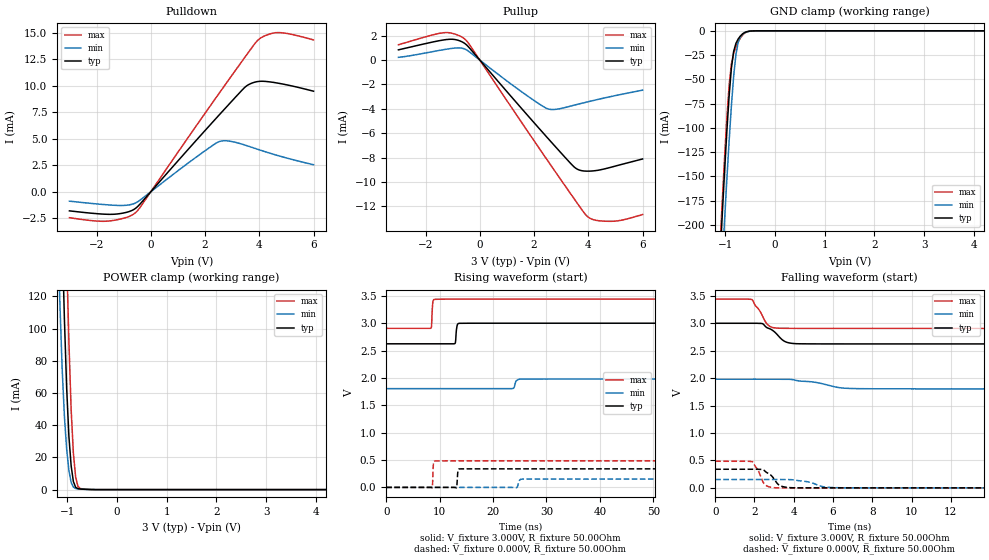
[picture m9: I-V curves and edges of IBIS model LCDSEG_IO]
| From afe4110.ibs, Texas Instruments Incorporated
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[Model]   LCDSEG_IO
Model_type   I/O
Vinl = 0.9V
Vinh = 2.1V
Vmeas = 1.500V
Cref = 25pF
|   typ   min   max
|   (NOM)   (WEAK)   (FAST)
C_comp   0.9946pF   0.9809pF   1.0463pF
[Model Spec]
Vinl   0.9V   0.594V   1.032V
Vinh   2.1V   1.386V   2.408V
[Voltage Range]   3.000V   1.980V   3.440V
[Temperature Range]   27.0   85.0   0.0
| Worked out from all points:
|   slope of the pulldown table from 0 to 0.45 V, typ, clamps not added: 342 ohm
|   slope of the pullup table from 0 to 0.45 V, typ, clamps not added: 385 ohm
|   GND clamp passes 1 mA (typ) near -0.57 V on its own axis
|   POWER clamp passes 1 mA (typ) near -0.81 V on its own axis
|   falling waveform, V_fixture 3.000V, R_fixture 50.00Ohm: 20-80 % time 803ps typ, 1.73ns min, 559ps max; typ from 3 V to 2.62 V
|   rising waveform, V_fixture 3.000V, R_fixture 50.00Ohm: 20-80 % time 203ps typ, 344ps min, 161ps max; typ from 2.62 V to 3 V
|   rising waveform, V_fixture 0.000V, R_fixture 50.00Ohm: 20-80 % time 139ps typ, 288ps min, 109ps max; typ from 0 V to 0.339 V
|   falling waveform, V_fixture 0.000V, R_fixture 50.00Ohm: 20-80 % time 535ps typ, 900ps min, 399ps max; typ from 0.339 V to 0 V
[Pulldown]
|   Voltage   I(typ)   I(min)   I(max)
-3V       -1.798mA   -884uA     -2.443mA
-1.598V   -2.122mA   -1.23mA    -2.769mA
-1.01V    -2.002mA   -1.288mA   -2.501mA
-603mV    -1.633mA   -1.101mA   -2.05mA
-376.9mV  -1.1mA     -754.7uA   -1.404mA
2.472V    7.106mA    4.676mA    9.115mA
2.834V    8.118mA    4.795mA    10.42mA
3.467V    9.847mA    4.407mA    12.67mA
3.965V    10.4mA     3.986mA    14.33mA
4.281V    10.39mA    3.726mA    14.78mA
4.688V    10.24mA    3.412mA    15.01mA
6V        9.481mA    2.549mA    14.32mA
[GND Clamp]
|   Voltage   I(typ)   I(min)   I(max)
-3V       -2.438A    -2.419A    -2.47A
-1.101V   -232.4mA   -281.6mA   -219.7mA
-1.055V   -187.1mA   -237.2mA   -173.3mA
-1.01V    -143.6mA   -194mA     -129.3mA
-964.8mV  -102.9mA   -152.5mA   -89.25mA
-919.6mV  -66.79mA   -113.3mA   -56.1mA
-874.4mV  -38.47mA   -77.46mA   -34.26mA
-829.1mV  -21.25mA   -47.02mA   -23.15mA
-783.9mV  -13.01mA   -24.69mA   -16.57mA
-738.7mV  -8.486mA   -11.97mA   -11.47mA
-603mV    -1.62mA    -1.923mA   -2.206mA
6V        0A         0A         0A
[Pullup]
|   Voltage   I(typ)   I(min)   I(max)
-3V       837uA      223uA      1.256mA
-1.327V   1.649mA    853.7uA    2.241mA
-919.6mV  1.683mA    980.9uA    2.13mA
-603mV    1.431mA    941.8uA    1.805mA
-376.9mV  979.2uA    661uA      1.255mA
2.472V    -6.315mA   -3.964mA   -8.145mA
2.834V    -7.212mA   -4.031mA   -9.311mA
3.513V    -8.822mA   -3.68mA    -11.47mA
3.965V    -9.104mA   -3.432mA   -12.81mA
4.281V    -9.056mA   -3.266mA   -13.13mA
4.869V    -8.765mA   -2.973mA   -13.21mA
6V        -8.106mA   -2.468mA   -12.66mA
[POWER Clamp]
|   Voltage   I(typ)   I(min)   I(max)
-3V       3.094A     2.811A     3.32A
-1.191V   277.9mA    163.8mA    401.2mA
-1.146V   216.5mA    115.6mA    333.9mA
-1.101V   158.6mA    75.42mA    268.1mA
-1.055V   106.3mA    45.57mA    204.8mA
-1.01V    63.3mA     25.24mA    145.1mA
-964.8mV  33.18mA    11.91mA    91.89mA
-919.6mV  14.78mA    4.503mA    49.65mA
-874.4mV  4.977mA    1.59mA     22.41mA
-829.1mV  1.449mA    719uA      7.81mA
-512.6mV  46.13uA    44.62uA    76.6uA
6V        0A         0A         0A
[Ramp]
R_load = 50.00Ohm
|   typ   min   max
dV/dt_r   203.508mV/138.836ps  91.470mV/287.777ps 290.967mV/109.240ps
dV/dt_f   225.897mV/803.247ps 105.264mV/1.734ns   320.282mV/559.231ps
[Falling Waveform]
V_fixture = 3.000V
V_fixture_min = 1.980V
V_fixture_max = 3.440V
R_fixture = 50.00Ohm
|   Time   V(typ)   V(min)   V(max)
0s        3V         1.98V      3.44V
1.86ns    3V         1.98V      3.434V
2.4ns     2.994V     1.98V      3.139V
2.69ns    2.911V     1.98V      2.969V
2.97ns    2.858V     1.98V      2.92V
3.4ns     2.704V     1.979V     2.909V
4.12ns    2.628V     1.959V     2.907V
6.42ns    2.624V     1.822V     2.906V
8.09ns    2.624V     1.806V     2.906V
100ns     2.624V     1.805V     2.906V
[Rising Waveform]
V_fixture = 3.000V
V_fixture_min = 1.980V
V_fixture_max = 3.440V
R_fixture = 50.00Ohm
|   Time   V(typ)   V(min)   V(max)
0s        2.624V     1.805V     2.906V
8.36ns    2.624V     1.805V     2.909V
8.73ns    2.624V     1.805V     3.379V
9.08ns    2.624V     1.805V     3.436V
12.85ns   2.628V     1.805V     3.44V
13.28ns   2.957V     1.805V     3.44V
13.7ns    2.998V     1.805V     3.44V
23.7ns    3V         1.807V     3.44V
25.31ns   3V         1.98V      3.44V
100ns     3V         1.98V      3.44V
[Rising Waveform]
V_fixture = 0.000V
V_fixture_min = 0.000V
V_fixture_max = 0.000V
R_fixture = 50.00Ohm
|   Time   V(typ)   V(min)   V(max)
0s        252.5nV    487nV      243.1nV
8.61ns    252.5nV    487.1nV    -8.246mV
8.84ns    252nV      487.1nV    427mV
9.14ns    248.9nV    487.1nV    483mV
13.13ns   -8.399mV   487nV      485mV
13.44ns   300.4mV    487nV      485mV
13.77ns   338.3mV    487nV      485mV
24.36ns   339.2mV    -4.759mV   484.9mV
25.7ns    339.2mV    152.4mV    484.9mV
100ns     339.2mV    152.5mV    484.9mV
[Falling Waveform]
V_fixture = 0.000V
V_fixture_min = 0.000V
V_fixture_max = 0.000V
R_fixture = 50.00Ohm
|   Time   V(typ)   V(min)   V(max)
0s        339.2mV    152.5mV    484.9mV
1.89ns    339.2mV    152.5mV    477.1mV
2.18ns    338.4mV    152.5mV    321.2mV
2.52ns    309.8mV    152.5mV    63.87mV
2.86ns    223.8mV    152.4mV    8.977mV
3.14ns    90.1mV     152.5mV    1.234mV
3.81ns    4.226mV    150.2mV    308.9uV
5.54ns    80.18uV    18.33mV    7.257uV
6.73ns    13.87uV    494.8uV    593.5nV
100ns     252.5nV    487nV      243.1nV
